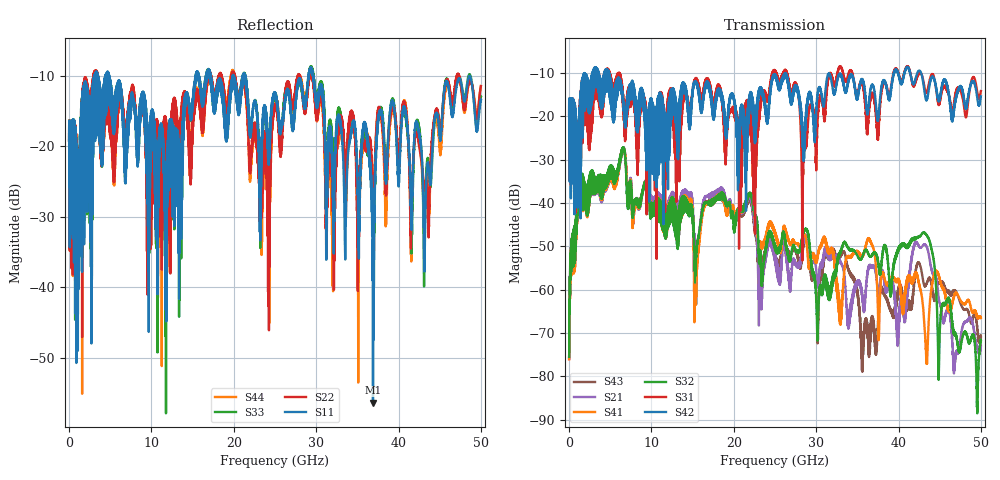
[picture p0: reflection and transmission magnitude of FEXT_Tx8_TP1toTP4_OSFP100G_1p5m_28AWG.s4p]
! Touchstone data
! Created: 27-Feb-2019 by IdEM 12 (12.1.0)
! COMMENTS
!  Created Wed Feb 27 09:43:39 2019
!  64 Port Network Data from SP1.SP block
!  freq  magS1_1  angS1_1  magS1_2  angS1_2  magS1_3  angS1_3  magS1_4  angS1_4
!  magS1_5  angS1_5  magS1_6  angS1_6  magS1_7  angS1_7  magS1_8  angS1_8
!  magS1_9  angS1_9  magS1_10  angS1_10  magS1_11  angS1_11  magS1_12  angS1_12
!  magS1_13  angS1_13  magS1_14  angS1_14  magS1_15  angS1_15  magS1_16  angS1_16
!  magS1_17  angS1_17  magS1_18  angS1_18  magS1_19  angS1_19  magS1_20  angS1_20
!  magS1_21  angS1_21  magS1_22  angS1_22  magS1_23  angS1_23  magS1_24  angS1_24
!  magS1_25  angS1_25  magS1_26  angS1_26  magS1_27  angS1_27  magS1_28  angS1_28
!  magS1_29  angS1_29  magS1_30  angS1_30  magS1_31  angS1_31  magS1_32  angS1_32
!  magS1_33  angS1_33  magS1_34  angS1_34  magS1_35  angS1_35  magS1_36  angS1_36
!  magS1_37  angS1_37  magS1_38  angS1_38  magS1_39  angS1_39  magS1_40  angS1_40
!  magS1_41  angS1_41  magS1_42  angS1_42  magS1_43  angS1_43  magS1_44  angS1_44
!  magS1_45  angS1_45  magS1_46  angS1_46  magS1_47  angS1_47  magS1_48  angS1_48
!  magS1_49  angS1_49  magS1_50  angS1_50  magS1_51  angS1_51  magS1_52  angS1_52
!  magS1_53  angS1_53  magS1_54  angS1_54  magS1_55  angS1_55  magS1_56  angS1_56
!  magS1_57  angS1_57  magS1_58  angS1_58  magS1_59  angS1_59  magS1_60  angS1_60
!  magS1_61  angS1_61  magS1_62  angS1_62  magS1_63  angS1_63  magS1_64  angS1_64
!  magS2_1  angS2_1  magS2_2  angS2_2  magS2_3  angS2_3  magS2_4  angS2_4
!  magS2_5  angS2_5  magS2_6  angS2_6  magS2_7  angS2_7  magS2_8  angS2_8
!  magS2_9  angS2_9  magS2_10  angS2_10  magS2_11  angS2_11  magS2_12  angS2_12
!  magS2_13  angS2_13  magS2_14  angS2_14  magS2_15  angS2_15  magS2_16  angS2_16
!  magS2_17  angS2_17  magS2_18  angS2_18  magS2_19  angS2_19  magS2_20  angS2_20
!  magS2_21  angS2_21  magS2_22  angS2_22  magS2_23  angS2_23  magS2_24  angS2_24
!  magS2_25  angS2_25  magS2_26  angS2_26  magS2_27  angS2_27  magS2_28  angS2_28
!  magS2_29  angS2_29  magS2_30  angS2_30  magS2_31  angS2_31  magS2_32  angS2_32
!  magS2_33  angS2_33  magS2_34  angS2_34  magS2_35  angS2_35  magS2_36  angS2_36
!  magS2_37  angS2_37  magS2_38  angS2_38  magS2_39  angS2_39  magS2_40  angS2_40
!  magS2_41  angS2_41  magS2_42  angS2_42  magS2_43  angS2_43  magS2_44  angS2_44
!  magS2_45  angS2_45  magS2_46  angS2_46  magS2_47  angS2_47  magS2_48  angS2_48
!  magS2_49  angS2_49  magS2_50  angS2_50  magS2_51  angS2_51  magS2_52  angS2_52
!  magS2_53  angS2_53  magS2_54  angS2_54  magS2_55  angS2_55  magS2_56  angS2_56
!  magS2_57  angS2_57  magS2_58  angS2_58  magS2_59  angS2_59  magS2_60  angS2_60
!  magS2_61  angS2_61  magS2_62  angS2_62  magS2_63  angS2_63  magS2_64  angS2_64
!  magS3_1  angS3_1  magS3_2  angS3_2  magS3_3  angS3_3  magS3_4  angS3_4
!  magS3_5  angS3_5  magS3_6  angS3_6  magS3_7  angS3_7  magS3_8  angS3_8
!  magS3_9  angS3_9  magS3_10  angS3_10  magS3_11  angS3_11  magS3_12  angS3_12
!  magS3_13  angS3_13  magS3_14  angS3_14  magS3_15  angS3_15  magS3_16  angS3_16
!  magS3_17  angS3_17  magS3_18  angS3_18  magS3_19  angS3_19  magS3_20  angS3_20
!  magS3_21  angS3_21  magS3_22  angS3_22  magS3_23  angS3_23  magS3_24  angS3_24
!  magS3_25  angS3_25  magS3_26  angS3_26  magS3_27  angS3_27  magS3_28  angS3_28
!  magS3_29  angS3_29  magS3_30  angS3_30  magS3_31  angS3_31  magS3_32  angS3_32
!  magS3_33  angS3_33  magS3_34  angS3_34  magS3_35  angS3_35  magS3_36  angS3_36
!  magS3_37  angS3_37  magS3_38  angS3_38  magS3_39  angS3_39  magS3_40  angS3_40
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# Hz S MA R 50
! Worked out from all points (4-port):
!   5000 points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, 10 MHz to 50 GHz, reference 50 ohm
!   strongest paths, dB at 10 MHz, 12.51 GHz, 25.01 GHz, 37.51 GHz, 50 GHz:
!     S42: -19.6, -16.2, -10.8, -21.0, -15.4
!     S31: -19.6, -16.6, -9.8, -25.4, -14.2
!     S32: -75.5, -43.8, -49.7, -53.3, -71.6
!     S41: -76.0, -43.5, -46.6, -65.5, -66.4
!     S21: -75.7, -41.7, -51.8, -60.1, -72.8
!     S43: -76.0, -42.1, -51.8, -67.2, -70.8
!   lowest |S11| = -56.3 dB at 36.9 GHz (marker M1), VSWR 1.00, Z = 50.1 + j0.121 ohm
!   |S11| at or under -10 dB: 4.861 GHz to 15.4 GHz (10.54 GHz wide, 104 % of centre); 21.38 GHz to 29.07 GHz (7.682 GHz wide, 30.5 % of centre); 29.66 GHz to end of sweep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
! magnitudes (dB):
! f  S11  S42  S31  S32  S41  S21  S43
! 10 MHz  -19.1  -19.6  -19.6  -75.5  -76.0  -75.7  -76.0
! 1.41 GHz  -19.7  -18.6  -18.5  -33.9  -34.3  -33.9  -34.1
! 6.58 GHz  -15.8  -16.9  -15.6  -27.3  -27.3  -27.2  -27.3
! 15.41 GHz  -9.7  -12.3  -11.3  -52.0  -57.6  -54.7  -59.7
! 21.9 GHz  -17.9  -15.5  -17.4  -37.7  -37.7  -38.4  -39.0
! 36.9 GHz  -56.3  -12.8  -14.9  -51.8  -50.3  -54.5  -67.4
! 50 GHz  -13.4  -15.4  -14.2  -71.6  -66.4  -72.8  -70.8
